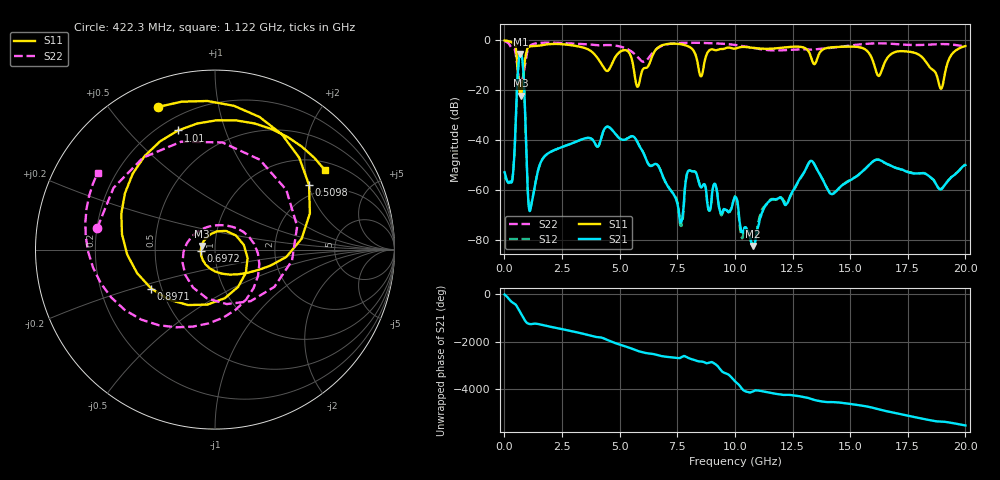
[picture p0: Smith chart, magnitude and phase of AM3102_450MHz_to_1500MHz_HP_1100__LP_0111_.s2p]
!Agilent Technologies,E8364B,MY43040894,A.07.50.67
!Agilent E8364B: A.07.50.67
!Date: Thursday, January 11, 2018 06:33:45
!Correction: S11(Full 2 Port(1,2))
!S21(Full 2 Port(1,2))
!S12(Full 2 Port(1,2))
!S22(Full 2 Port(1,2))
!S2P File: Measurements: S11, S21, S12, S22:
# Hz S  dB  R 50
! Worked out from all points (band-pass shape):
!   1601 points, 10 MHz to 20 GHz, reference 50 ohm
!   highest |S21| = -5.44 dB at 697.2 MHz (marker M1); lowest = -82.3 dB at 10.78 GHz (marker M2)
!   |S21| within 3 dB of the highest: 621.9 MHz to 788.2 MHz (166.3 MHz wide, 23.6 % of centre)
!   lowest |S11| = -22.2 dB at 709.6 MHz (marker M3), VSWR 1.17, Z = 43 + j1.8 ohm
!   |S11| at or under -10 dB: 5.585 GHz to 6.26 GHz (675.1 MHz wide, 11.4 % of centre); 16.05 GHz to 16.45 GHz (400.2 MHz wide, 2.46 % of centre); 18.38 GHz to 19.2 GHz (810.9 MHz wide, 4.32 % of centre)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
!   |S22| runs from -17.5 to -0.4 dB; largest |S21 - S12| = 0.00083
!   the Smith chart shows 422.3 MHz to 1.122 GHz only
!   S11 on the Smith chart (normalised r, x): 422.3 MHz: 0.11, +0.67; 509.8 MHz: 1.68, +2.02; 697.2 MHz: 0.85, -0.01; 897.1 MHz: 0.44, -0.23; 1.01 GHz: 0.27, +0.70; 1.122 GHz: 1.24, +2.56
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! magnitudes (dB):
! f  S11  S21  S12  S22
! 10 MHz  -0.1  -52.8  -54.8  -0.4
! 422.3 MHz  -1.4  -47.4  -47.6  -3.5
! 509.8 MHz  -3.9  -28.0  -28.0  -6.4
! 697.2 MHz  -22.0  -5.4  -5.4  -17.5
! 709.6 MHz  -22.2  -5.5  -5.5  -17.5
! 897.1 MHz  -7.6  -28.4  -28.3  -9.7
! 1.01 GHz  -3.2  -59.1  -59.0  -3.9
! 1.122 GHz  -2.4  -68.0  -67.8  -2.1
! 1.709 GHz  -1.8  -46.8  -46.8  -1.0
! 3.346 GHz  -2.7  -39.7  -39.7  -1.5
! 5.782 GHz  -18.6  -41.0  -40.9  -6.7
! 6.682 GHz  -2.8  -50.3  -50.3  -3.0
! 7.669 GHz  -1.6  -72.8  -74.3  -1.1
! 8.031 GHz  -2.6  -52.1  -52.0  -1.0
! 8.531 GHz  -14.5  -58.9  -58.6  -1.0
! 10.01 GHz  -3.4  -62.7  -62.4  -1.9
! 10.78 GHz  -3.0  -82.3  -82.3  -3.0
! 13.34 GHz  -7.9  -48.3  -48.2  -3.7
! 14.22 GHz  -2.8  -61.6  -61.2  -3.0
! 16.68 GHz  -6.4  -49.8  -49.8  -1.3
! 18.94 GHz  -19.4  -59.6  -59.4  -1.5
! 20 GHz  -2.3  -50.0  -49.7  -2.4
